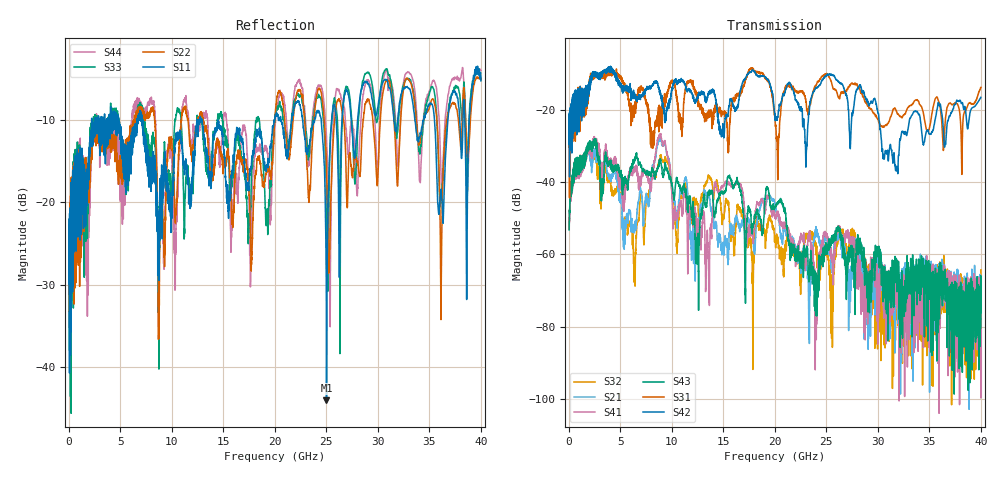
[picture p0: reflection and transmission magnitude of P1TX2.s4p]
!Agilent Technologies,N5245A,MY49151084,A.09.20.08
!Agilent N5245A: A.09.20.08
!Date: Thursday, March 01, 2012 14:12:48
!Correction: S11(Full 4 Port(1,2,3,4))
!S12(Full 4 Port(1,2,3,4))
!S13(Full 4 Port(1,2,3,4))
!S14(Full 4 Port(1,2,3,4))
!S21(Full 4 Port(1,2,3,4))
!S22(Full 4 Port(1,2,3,4))
!S23(Full 4 Port(1,2,3,4))
!S24(Full 4 Port(1,2,3,4))
!S31(Full 4 Port(1,2,3,4))
!S32(Full 4 Port(1,2,3,4))
!S33(Full 4 Port(1,2,3,4))
!S34(Full 4 Port(1,2,3,4))
!S41(Full 4 Port(1,2,3,4))
!S42(Full 4 Port(1,2,3,4))
!S43(Full 4 Port(1,2,3,4))
!S44(Full 4 Port(1,2,3,4))
!S4P File: Measurements: <S11,S12,S13,S14>,
!<S21,S22,S23,S24>,
!<S31,S32,S33,S34>,
!<S41,S42,S43,S44>:
# Hz S  dB  R 50
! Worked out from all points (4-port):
!   3996 points, 50 MHz to 40 GHz, reference 50 ohm
!   strongest paths, dB at 50 MHz, 10.04 GHz, 20.03 GHz, 30.02 GHz, 40 GHz:
!     S42: -23.6, -14.0, -22.1, -21.0, -16.5
!     S31: -25.6, -12.2, -23.0, -22.6, -13.8
!     S43: -53.2, -40.8, -47.0, -58.9, -76.1
!     S41: -51.7, -44.0, -49.4, -73.0, -81.8
!     S21: -51.5, -43.9, -46.1, -60.1, -67.7
!     S32: -52.6, -43.3, -55.9, -69.7, -64.3
!   lowest |S11| = -44.1 dB at 25.02 GHz (marker M1), VSWR 1.01, Z = 50.6 + j0.0263 ohm
!   |S11| at or under -10 dB: start of sweep to 2.237 GHz; 7.17 GHz to 12.47 GHz (5.299 GHz wide, 54 % of centre); 12.96 GHz to 19.93 GHz (6.967 GHz wide, 42.4 % of centre)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
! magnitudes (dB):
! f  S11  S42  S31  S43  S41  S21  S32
! 50 MHz  -24.3  -23.6  -25.6  -53.2  -51.7  -51.5  -52.6
! 6.38 GHz  -12.2  -16.8  -19.5  -33.7  -36.6  -52.8  -62.1
! 8.82 GHz  -20.9  -15.0  -23.9  -34.3  -26.8  -28.2  -33.8
! 13.48 GHz  -14.6  -16.6  -21.7  -43.6  -55.9  -43.8  -39.2
! 25.02 GHz  -44.1  -10.6  -9.9  -58.8  -54.3  -54.2  -58.5
! 31.79 GHz  -11.4  -36.0  -20.3  -61.1  -66.3  -72.6  -72.6
! 40 GHz  -5.3  -16.5  -13.8  -76.1  -81.8  -67.7  -64.3
